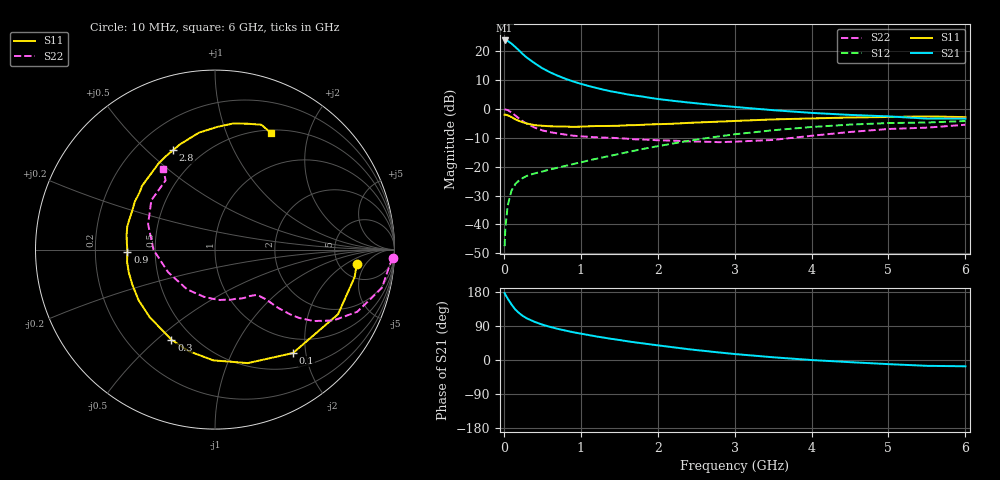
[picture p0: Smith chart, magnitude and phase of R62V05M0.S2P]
! SIEMENS Small Signal Semiconductors
! BFR193
! Si NPN RF Bipolar Junction Transistor in SOT23
! VCE = 2 V  IC = 5 mA
! Common Emitter S-Parameters:  May  1996
# GHz  S  MA  R  50
!  f  S11  S21  S12  S22
! GHz  MAG  ANG  MAG  ANG  MAG  ANG  MAG  ANG
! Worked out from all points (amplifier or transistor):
!   36 points, 10 MHz to 6 GHz, reference 50 ohm
!   highest |S21| = 23.7 dB at 10 MHz (marker M1)
!   |S21| within 3 dB of that: start of sweep to 179 MHz
!   unconditionally stable (mu >= 1): 874.6 MHz to 2.052 GHz
!   at 250 MHz: K = 0.43, MSG = 21.4 dB, |S12| = -23.9 dB
!   at 1.4 GHz: K = 1.07, MAG = 9.5 dB, |S12| = -16.2 dB
!   at 6 GHz: K = 0.97, MSG = 0.4 dB, |S12| = -4.2 dB
!   lowest NFmin = 1.20 dB at 450 MHz
!   S11 on the Smith chart (normalised r, x): 10 MHz: 7.32, -3.19; 100 MHz: 0.73, -1.77; 300 MHz: 0.38, -0.56; 900 MHz: 0.34, -0.01; 2.8 GHz: 0.35, +0.61; 6 GHz: 0.54, +1.45
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0.01  0.7945 -5.8  15.31 176.6  0.0042 86.8  0.9912 -2.7
0.02  0.7927 -11.2  15.2 172.6  0.0087 87.1  0.9772 -5.1
0.05  0.7744 -27.7  15 162.0  0.0212 76.7  0.9542 -12.9
0.1  0.7217 -53.0  13.52 146.4  0.0384 65.3  0.865 -23.6
0.15  0.6582 -73.9  11.75 133.1  0.0501 57.6  0.7691 -30.9
0.2  0.6171 -90.9  10.23 123.5  0.0581 52.3  0.6788 -35.9
0.25  0.584 -104.8  8.79 115.9  0.064 49.0  0.6062 -39.0
0.3  0.5571 -115.9  7.712 109.8  0.0694 47.7  0.5555 -40.7
0.4  0.5236 -134.1  6.187 100.7  0.0763 46.4  0.4752 -42.8
0.5  0.5104 -146.6  5.058 93.4  0.0824 46.9  0.4243 -43.7
0.6  0.5005 -156.9  4.306 87.5  0.0896 47.8  0.3965 -44.3
0.7  0.497 -165.1  3.758 82.2  0.0958 49.4  0.3758 -45.3
0.9  0.488 -178.5  2.987 73.4  0.1108 52.7  0.3438 -47.6
1.1  0.4993 170.5  2.499 66.0  0.1278 55.3  0.3287 -51.3
1.3  0.5057 161.2  2.147 59.0  0.1462 56.9  0.3179 -55.4
1.6  0.5208 149.2  1.789 49.6  0.1773 58.0  0.3053 -63.6
2.2  0.5535 129.8  1.381 33.6  0.2517 55.9  0.282 -84.6
2.8  0.6018 112.7  1.143 19.9  0.335 49.5  0.2657 -114.0
3.5  0.6573 97.9  0.951 7.2  0.427 38.6  0.2902 -154.4
4.5  0.7099 81.8  0.787 -5.7  0.5349 21.9  0.3988 159.2
5.5  0.7422 69.6  0.679 -15.4  0.5806 5.0  0.4738 125.5
6  0.7207 64.4  0.679 -16.6  0.6169 0.1  0.5314 122.8
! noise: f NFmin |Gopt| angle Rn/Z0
0.45  1.2  0.26  102  0.14
0.9  1.25  0.38  145  0.12
1.8  2.05  0.56  -161  0.12
